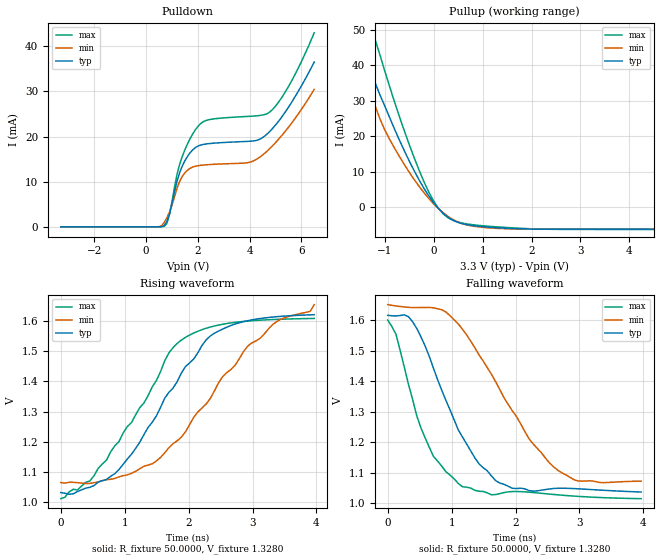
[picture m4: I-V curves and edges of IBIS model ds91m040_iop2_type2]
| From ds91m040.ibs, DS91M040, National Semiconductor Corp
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|   Model ds91m040_iop2_type2
[Model] ds91m040_iop2_type2
Model_type I/O
Polarity   Non-Inverting
Vinl = 0.05
Vinh = 0.15
Vmeas =  1.56V
Rref =   50.0000
Vref =   1.56V
C_comp   7.359p   6.991p  7.743p
[Model Spec]
S_overshoot_high   3.8   3.8   3.8
S_overshoot_low   -1.4   -1.4   -1.4
[Temperature Range]   25.0000   85.0000   -40.0000
[Voltage Range]   3.3000V   3.0000V   3.6000V
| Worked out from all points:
|   slope of the pullup table from 0 to 0.495 V, typ, clamps not added: 89.8 ohm
|   rising waveform, R_fixture 50.0000, V_fixture 1.3280: 20-80 % time 1.1ns typ, 1.37ns min, 1.01ns max; typ from 1.03 V to 1.62 V
|   falling waveform, R_fixture 50.0000, V_fixture 1.3280: 20-80 % time 738ps typ, 1.02ns min, 589ps max; typ from 1.62 V to 1.04 V
[Pulldown]
|Voltage   I(typ)   I(min)   I(max)
-3.3V     -16.03uA   -15.03uA   -17.07uA
500mV     -1.779uA   19.11uA    -4.505uA
700mV     266.1uA    947.9uA    95.95uA
900mV     2.789mA    3.225mA    2.636mA
1.2V      10.22mA    8.651mA    11.74mA
1.4V      13.49mA    11.17mA    15.63mA
2V        17.87mA    13.53mA    22.22mA
2.5V      18.47mA    13.8mA     23.81mA
4V        18.95mA    14.28mA    24.48mA
4.8V      21.23mA    17.43mA    25.52mA
5.6V      27.34mA    22.77mA    32.05mA
6.5V      36.5mA     30.45mA    42.97mA
[Pullup]
|Voltage   I(typ)   I(min)   I(max)
-3.3V     175.6mA    142.3mA    190.5mA
-1.7V     63.38mA    52.81mA    76.23mA
-1.6V     56.8mA     47.64mA    68.59mA
-1.5V     50.5mA     42.58mA    62.09mA
-1.3V     39.51mA    33.04mA    51.53mA
-1.2V     35.24mA    28.74mA    47.34mA
-900mV    25.28mA    19.17mA    33.99mA
-200mV    5.404mA    4.186mA    7.28mA
100mV     -330.9uA   -343uA     -296.8uA
500mV     -4.222mA   -4.121mA   -4.112mA
1.6V      -5.915mA   -6.038mA   -5.727mA
6.5V      -6.152mA   -6.146mA   -6.187mA
[Ramp]
| variable   typ   min   max
dV/dt_r  0.3571/1.190n   0.3519/1.440n   0.3593/1.070n
dV/dt_f  0.3557/0.812n   0.3514/1.110n   0.3588/0.645n
R_load = 50.00
[Rising Waveform]
R_fixture= 50.0000
V_fixture= 1.3280
V_fixture_min= 1.3569
V_fixture_max= 1.3117
|time   V(typ)   V(min)   V(max)
0s        1.032V     1.065V     1.011V
455ps     1.049V     1.062V     1.07V
845ps     1.094V     1.078V     1.186V
1.43ns    1.264V     1.127V     1.381V
1.69ns    1.363V     1.18V      1.494V
1.885ns   1.427V     1.215V     1.537V
2.275ns   1.538V     1.325V     1.576V
2.6ns     1.58V      1.43V      1.592V
3.315ns   1.613V     1.589V     1.605V
3.965ns   1.621V     1.654V     1.609V
[Falling Waveform]
R_fixture= 50.0000
V_fixture= 1.3280
V_fixture_min= 1.3569
V_fixture_max= 1.3117
|time   V(typ)   V(min)   V(max)
0s        1.617V     1.652V     1.601V
130ps     1.615V     1.647V     1.554V
325ps     1.612V     1.643V     1.39V
650ps     1.482V     1.643V     1.184V
1.17ns    1.218V     1.571V     1.054V
1.755ns   1.066V     1.373V     1.032V
2.21ns    1.042V     1.212V     1.037V
2.6ns     1.049V     1.119V     1.029V
2.99ns    1.047V     1.073V     1.023V
3.965ns   1.037V     1.072V     1.015V
